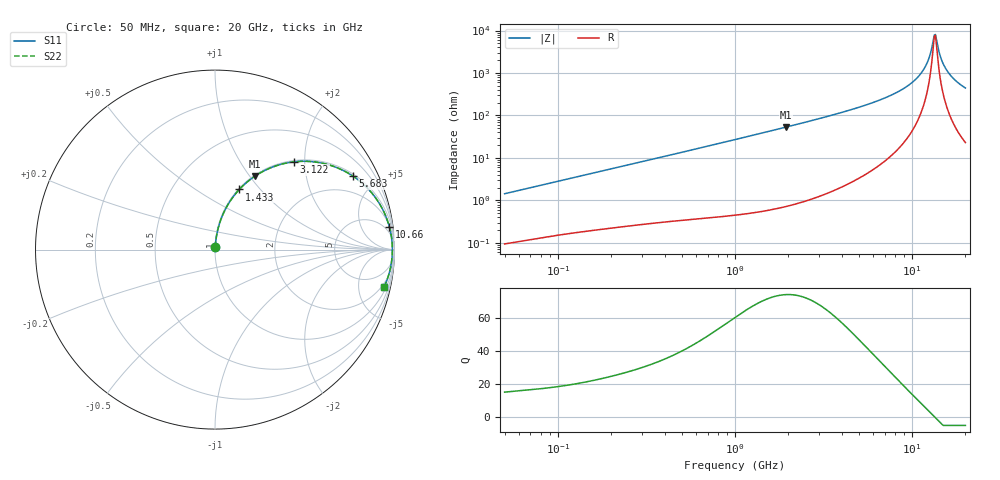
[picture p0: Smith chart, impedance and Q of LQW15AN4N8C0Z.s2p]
!Murata Part Number: LQW15AN4N8C0Z
!These Parameters are Measured in Series Mode Connection
!  o--[Z]--o
!Port1  Port2
!  o-------o
!Freq. Start=50[MHz] Stop=20[GHz], 401[Steps]
# Hz S RI R 50
!Freq.(Hz) S11(Real) S11(Imag) S21(Real) S21(Imag) S12(Real) S12(Imag) S22(Real) S22(Imag)
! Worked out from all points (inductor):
!   401 points, 50 MHz to 20 GHz, reference 50 ohm
!   read as one part in series: L = 4.53 nH near 51.52 MHz
!   highest Q = 74.2 at 1.933 GHz (marker M1), where L = 4.37 nH
!   self-resonance near 13.35 GHz
!   S11 on the Smith chart (normalised r, x): 50 MHz: 1.00, +0.03; 1.433 GHz: 1.01, +0.78; 3.122 GHz: 1.03, +1.77; 5.683 GHz: 1.09, +3.71; 10.66 GHz: 2, +15; 20 GHz: 1.46, -8.87
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5e7  0.00115 0.0143  0.9989 -0.0143  0.9989 -0.0143  0.00115 0.0143
1.364002e8  0.00324 0.0377  0.9968 -0.0377  0.9968 -0.0377  0.00324 0.0377
3.721004e8  0.013 0.0996  0.987 -0.0996  0.987 -0.0996  0.013 0.0996
1e9  0.0719 0.2502  0.9281 -0.2502  0.9281 -0.2502  0.0719 0.2502
1.432596e9  0.1353 0.3351  0.8647 -0.3351  0.8647 -0.3351  0.1353 0.3351
1.932977e9  0.2227 0.4094  0.7773 -0.4094  0.7773 -0.4094  0.2227 0.4094
2.728004e9  0.3705 0.4759  0.6295 -0.4759  0.6295 -0.4759  0.3705 0.4759
3.121702e9  0.4408 0.489  0.5592 -0.489  0.5592 -0.489  0.4408 0.489
4.212059e9  0.6094 0.4789  0.3906 -0.4789  0.3906 -0.4789  0.6094 0.4789
5.683258e9  0.7697 0.409  0.2303 -0.409  0.2303 -0.409  0.7697 0.409
7.442007e9  0.8837 0.3032  0.1163 -0.3032  0.1163 -0.3032  0.8837 0.3032
9.178299e9  0.9445 0.2026  0.0555 -0.2026  0.0555 -0.2026  0.9445 0.2026
1.066139e10  0.9721 0.125  0.0279 -0.125  0.0279 -0.125  0.9721 0.125
1.201863e10  0.9844 0.0611  0.0156 -0.0611  0.0156 -0.0611  0.9844 0.0611
1.257102e10  0.9869 0.037  0.0131 -0.037  0.0131 -0.037  0.9869 0.037
1.314879e10  0.9881 0.0127  0.0119 -0.0127  0.0119 -0.0127  0.9881 0.0127
1.354865e10  0.9883 -0.00349  0.0117 0.00349  0.0117 0.00349  0.9883 -0.00349
1.375312e10  0.9882 -0.0116  0.0118 0.0116  0.0118 0.0116  0.9882 -0.0116
1.460232e10  0.9864 -0.0439  0.0136 0.0439  0.0136 0.0439  0.9864 -0.0439
1.573793e10  0.9812 -0.0842  0.0188 0.0842  0.0188 0.0842  0.9812 -0.0842
1.747767e10  0.9682 -0.1398  0.0318 0.1398  0.0318 0.1398  0.9682 -0.1398
2e10  0.942 -0.2093  0.058 0.2093  0.058 0.2093  0.942 -0.2093
